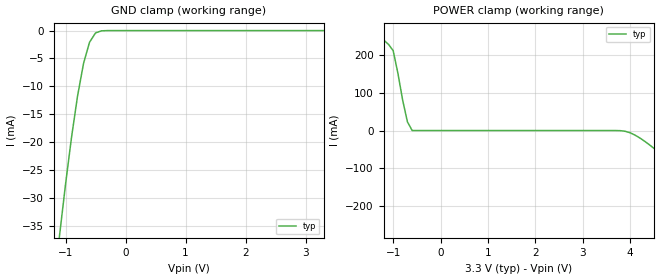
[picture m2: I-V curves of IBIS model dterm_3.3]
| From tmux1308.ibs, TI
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| dterm_3.3
[Model]   dterm_3.3
Model_type   Terminator
|   typ   min   max
C_comp   1.008417e-11   NA   NA
[Voltage Range]   3.3   NA   NA
[Temperature Range]   27   NA   NA
[Power Clamp Reference]   3.3   NA   NA
[GND Clamp Reference]   0   NA   NA
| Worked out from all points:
|   GND clamp passes 1 mA (typ) near -0.53 V on its own axis
|   POWER clamp passes 1 mA (typ) near -0.60 V on its own axis
[GND Clamp]
|   Voltage   I(typ)   I(min)   I(max)
-6.6V     -37.87kA   NA         NA
-1.1V     -36.75mA   NA         NA
-900mV    -19.13mA   NA         NA
-800mV    -11.75mA   NA         NA
-700mV    -5.894mA   NA         NA
-600mV    -2.091mA   NA         NA
-500mV    -418.9uA   NA         NA
-400mV    -46.02uA   NA         NA
-300mV    -3.126uA   NA         NA
3.3V      1.528nA    NA         NA
[POWER Clamp]
|   Voltage   I(typ)   I(min)   I(max)
-3.3V     443.5mA    NA         NA
-1.6V     276.2mA    NA         NA
-1.2V     238.3mA    NA         NA
-1V       210.6mA    NA         NA
-700mV    23.04mA    NA         NA
-600mV    83.61uA    NA         NA
4V        -5.894mA   NA         NA
4.4V      -36.75mA   NA         NA
5.1V      -112.4mA   NA         NA
6.1V      -233.5mA   NA         NA
6.3V      -329.9mA   NA         NA
6.6V      -1.138kA   NA         NA
